DATA_BLOCK DB 22
TITLE =BLOCK DATA FOR NUMBER PAGE OP_37
//
//
AUTHOR : Esposito
FAMILY : EGAL_srl
NAME : PAGE_OP
VERSION : 0.1


  STRUCT
   Page_OP_370 : INT ;
   Page_OP_371 : INT ;
   Page_OP_372 : INT ;
   Page_OP_373 : INT ;
   Page_OP_374 : INT ;
  END_STRUCT ;
BEGIN
   Page_OP_370 := 0;
   Page_OP_371 := 0;
   Page_OP_372 := 0;
   Page_OP_373 := 0;
   Page_OP_374 := 0;
END_DATA_BLOCK

